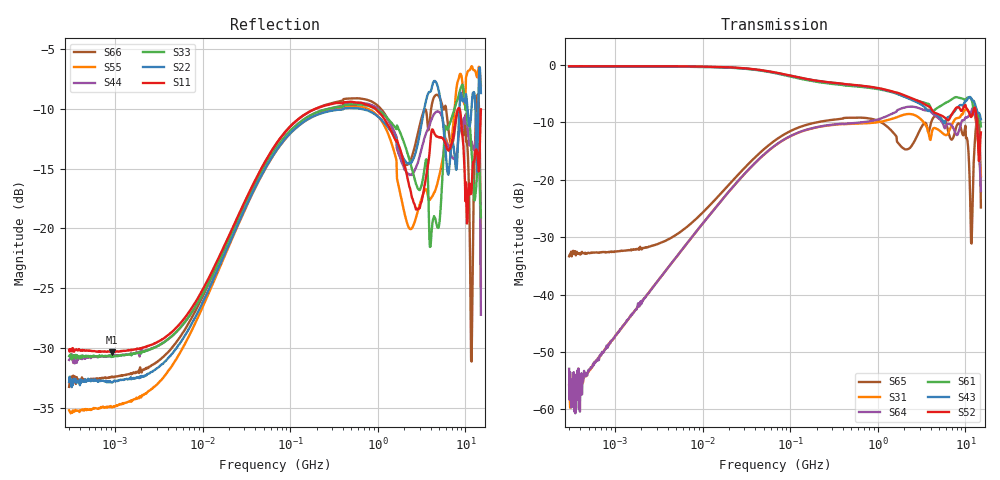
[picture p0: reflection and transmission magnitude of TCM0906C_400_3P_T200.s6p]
! S-Parameter Data Generated by TDK Corporation
! Copyright(C) 2023 TDK Corporation.
! All Rights Reserved.
! TDK P/N: TCM0906C-400-3P-T200 (Common Mode Filter)
! Property: |Zc|=40ohm at 100MHz
! Size(LxWxT): 0.875x0.65x0.4mm
! Model Type: s6p (Touchstone File Format Version 1.0)
! Frequency: DC=Yes Start=0.3MHz Stop=15000MHz 802points Log-sweep
! Model Generated on June 19, 2023
! Port Assignments:
!  1 ---@@@--- 6
!  2 ---@@@--- 5
!  3 ---@@@--- 4
! Applicable Conditions:
!  Temperature = 25 degC
!  DC Bias Current = 0 A
!  Small Signal Operation
! Terms and conditions regarding TDK Simulation Models
! (1)This simulation model is being provided solely for informational purposes. Please refer to the specifications of the products in terms of detailed characteristics of such products.
! (2)In no event shall TDK Corporation of any of its subsidiaries be liable for any loss or damage arising, directly or indirectly,
!  From any information contained in this simulation model, including, but not limited to loss or damages arising from any inaccuracies, omissions or errors in connection with such information.
! (3)Any and all copyrights on this simulation model are owned by TDK Corporation.
!  Duplication or redistribution of this simulation model without prior written permission from TDK Corporation is prohibited.
! (4)This simulation model is subject to any modification or change without any prior notice.
! (5)Neither TDK Corporation nor any of its subsidiaries shall make any warranty, express or implied,
!  Including but not limited to the correctness, implied warranties of merchantability and fitness for a particular purpose with respect to this simulation models.
! (6)The use of this simulation model shall be deemed to have consented to the terms and conditions hereof.
# Hz S MA R 50
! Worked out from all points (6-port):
!   801 points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, 300 kHz to 15 GHz, reference 50 ohm
!   strongest paths, dB at 300 kHz, 4.486 MHz, 67.08 MHz, 1.003 GHz, 15 GHz:
!     S52: -0.2, -0.2, -1.3, -4.0, -11.7
!     S43: -0.3, -0.3, -1.3, -4.0, -9.5
!     S61: -0.3, -0.3, -1.4, -4.2, -10.7
!     S64: -52.9, -34.4, -14.0, -9.5, -22.0
!     S31: -55.8, -34.4, -14.1, -10.0, -19.4
!     S65: -33.3, -30.0, -13.1, -9.7, -24.8
!   lowest |S11| = -30.3 dB at 921.8 kHz (marker M1), VSWR 1.06, Z = 53.1 + j0.319 ohm
!   |S11| at or under -10 dB: start of sweep to 195.9 MHz; 933.6 MHz to 8.27 GHz (7.336 GHz wide, 159 % of centre); 8.537 GHz to end of sweep
